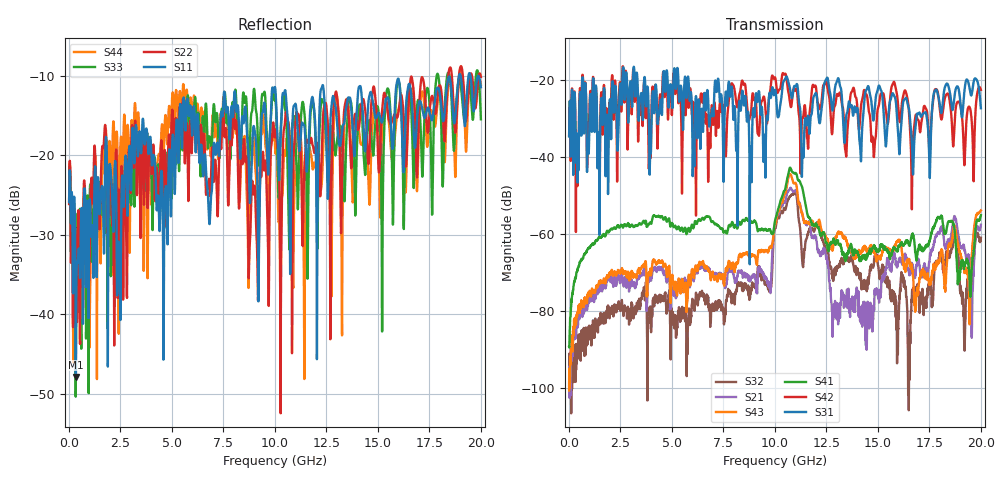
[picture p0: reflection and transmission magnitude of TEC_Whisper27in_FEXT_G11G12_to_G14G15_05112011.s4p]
! Tyco Electronics
! G11G12-G14G15_FEXT
!! PART DESCRIPTION: Whisper 27in Megtron 6 VLP-HVLP-VLP Channel Model, bulkhead 2.4mm test pts
!! MODEL DESCRIPTION: System 4-port S-parameter
!! MODEL STATUS: Measured
!! MODEL GEOMETRY: Channel Model
!! MODEL FREQUENCY RANGE: DC to 20.000 GHz in 10.000 MHz frequency steps
!! MODEL EDGE RATE LIMITATION: 25.00 ps (Using conservative 0.5/Fmax rule of thumb)
!! TIME-DOMAIN TRANSFORM CAUTIONS:
!! 1.) Do not simulate transient edge rates faster than the number listed above.  Edge rates faster than this number
!!  contain significant spectral content at frequencies above the model's highest frequency.
!! 2.) Even when simulating edge rates that are slower than the number listed above, be aware that the best time
!!  resolution possible with a direct iFFT is (1 / 2Fmax).  As a result, time resolution is typically not adequate
!!  for most time-domain simulations unless tricks such as windowing are used to minimize leakage and aliasing.
!! 3.) Because the model has a uniform frequency step, a direct iFFT will result in an impulse that that has a time
!!  length given by either (1 / Fstep) or (1 / 2Fstep), depending on the transform being used.  Care has been taken
!!  in selecting the frequency step to ensure a settled impulse response for the model.  Therefore, convolution with
!!  the model's impulse response should present no issues.  However, if directly concatenating s-parameter models
!!  in the frequency domain a user must either interpolate necessary interim frequencies or complete impulse response
!!  zero-padding.  Impulse response zero-padding is more difficult, but more accurate.
!! PORT DEFINITIONS:
!! Port  1  ----->  Side A  G11  G14  Side B  <-----  Port  2
!! Port  3  ----->  Side A  G12  G15  Side B  <-----  Port  4
! Point-to-Point link (differential)  !
! Connectors:  !
!  1: STRADA Whisper  !
! Materials:  !
!  Backplane: Megtron-6 HVLP  !
!  Daughtercard: Megtron-6 VLP  !
! Stack-up:  !
!  Backplane: 20 layers, 200mil thick  !
!  Daughtercard: 14 layers, 110mil thick  !
! Trace Length:  !
!  Backplane: 17in  !
!  Daightercards: 5in  !
! Trace Width:  !
!  Backplane: 8-13-8 mils  !
!  Daughtercards: 6-9-6 mils  !
! Geometry:  !
!  Backplane: Stripline  !
!  Daughtercards: Stripline  !
! Freq. Range: 0 GHz - 20 GHz  !
! Note1: non-mixed-mode s-parameters  !
! Note2: channel includes 2.4mm test points  !
! Created Wed May 11 14:43:36 2011
! 4 Port Network Data from SP1.SP block
! freq  magS11  angS11  magS12  angS12  magS13  angS13  magS14  angS14
!  magS21  angS21  magS22  angS22  magS23  angS23  magS24  angS24
!  magS31  angS31  magS32  angS32  magS33  angS33  magS34  angS34
!  magS41  angS41  magS42  angS42  magS43  angS43  magS44  angS44
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# hz S ma R 50
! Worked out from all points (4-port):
!   2000 points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, 10 MHz to 20 GHz, reference 50 ohm
!   strongest paths, dB at 10 MHz, 5.01 GHz, 10.01 GHz, 15.01 GHz, 20 GHz:
!     S31: -34.6, -25.9, -22.5, -22.0, -27.2
!     S42: -34.4, -27.9, -19.2, -27.2, -22.5
!     S41: -89.2, -57.0, -56.3, -64.0, -55.0
!     S43: -100.5, -70.9, -57.6, -65.8, -53.8
!     S21: -99.2, -73.1, -57.1, -76.4, -57.5
!     S32: -98.7, -80.0, -58.5, -68.1, -60.9
!   lowest |S11| = -47.8 dB at 340 MHz (marker M1), VSWR 1.01, Z = 50.2 + j0.341 ohm
!   |S11| at or under -10 dB: start of sweep to 18.94 GHz; 19.02 GHz to 19.4 GHz (383.3 MHz wide, 2 % of centre); 19.49 GHz to 19.86 GHz (368.8 MHz wide, 1.87 % of centre)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
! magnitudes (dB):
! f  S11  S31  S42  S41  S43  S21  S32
! 10 MHz  -25.9  -34.6  -34.4  -89.2  -100.5  -99.2  -98.7
! 340 MHz  -47.8  -41.4  -59.4  -71.0  -83.3  -84.7  -88.5
! 9.72 GHz  -19.2  -23.8  -24.3  -58.7  -63.6  -73.4  -73.8
! 10.73 GHz  -31.2  -22.1  -25.6  -42.7  -44.3  -48.1  -50.0
! 13.04 GHz  -16.7  -19.8  -23.7  -61.6  -59.6  -80.7  -68.1
! 16.85 GHz  -17.6  -30.5  -28.9  -65.9  -78.5  -68.7  -75.1
! 20 GHz  -11.4  -27.2  -22.5  -55.0  -53.8  -57.5  -60.9
